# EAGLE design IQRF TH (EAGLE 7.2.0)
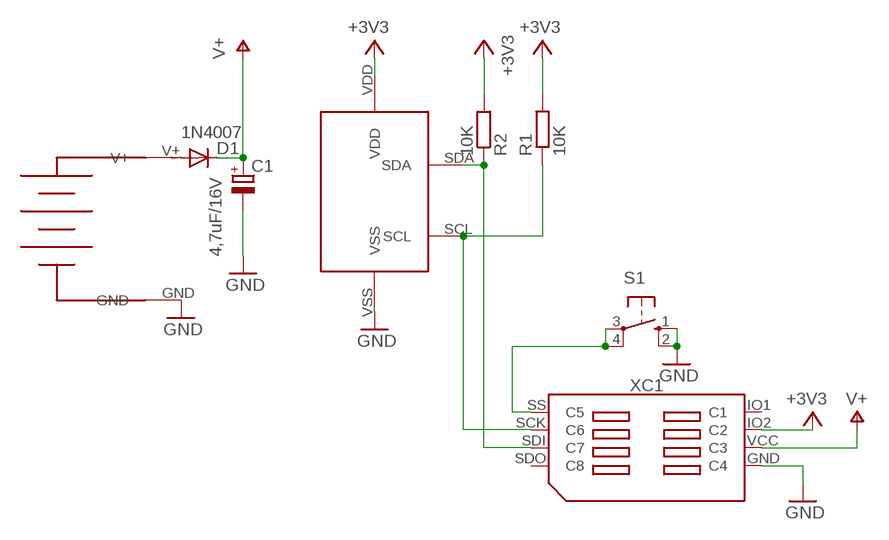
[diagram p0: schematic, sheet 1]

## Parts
3XAA1,5V  3AA  [3AA]
C1  4,7uF/16V  CPOL-EUE2,5-6E  [E2,5-6E]
D1  1N4007  DIODE-DO34-7  [DO34-7]
R1  10K  R-EU_0207/7  [0207/7]
R2  10K  R-EU_0207/7  [0207/7]
S1  10-XX  [B3F-10XX]
U$1  BOB21  [BOB21]
XC1  SIM8X_KON-SIM02  [SIM_02]

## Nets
+3V3: R1.2 R2.2 U$1.VDD XC1.IO2(C2)
GND: 3XAA1,5V.GND C1.- S1.1(S) S1.2(S1) U$1.VSS XC1.GND(C4)
N$1: 3XAA1,5V.V+ D1.A
N$2: R1.1 U$1.SCL XC1.SCK(C6)
N$3: S1.3(P) S1.4(P1) XC1.SS(C5)
N$4: R2.1 U$1.SDA XC1.SDI(C7)
V+: C1.+ D1.C
Unconnected: XC1.IO1(C1) XC1.SDO(C8) XC1.VCC(C3)

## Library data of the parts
3XAA1,5V = battery:3AA
C1 = rcl:CPOL-EU: POLARIZED CAPACITOR, European symbol
D1 = diode:DIODE-: DIODE
R1 R2 = rcl:R-EU_: RESISTOR, European symbol
S1 = switch-omron:10-XX: OMRON SWITCH; MPN: B3F-1000; OC_FARNELL: 176432; OC_NEWARK: 36M3542
U$1 = sinserion:BOB21
XC1 = KON-SIM-02_150624:SIM8X_KON-SIM: KON-SIM-02

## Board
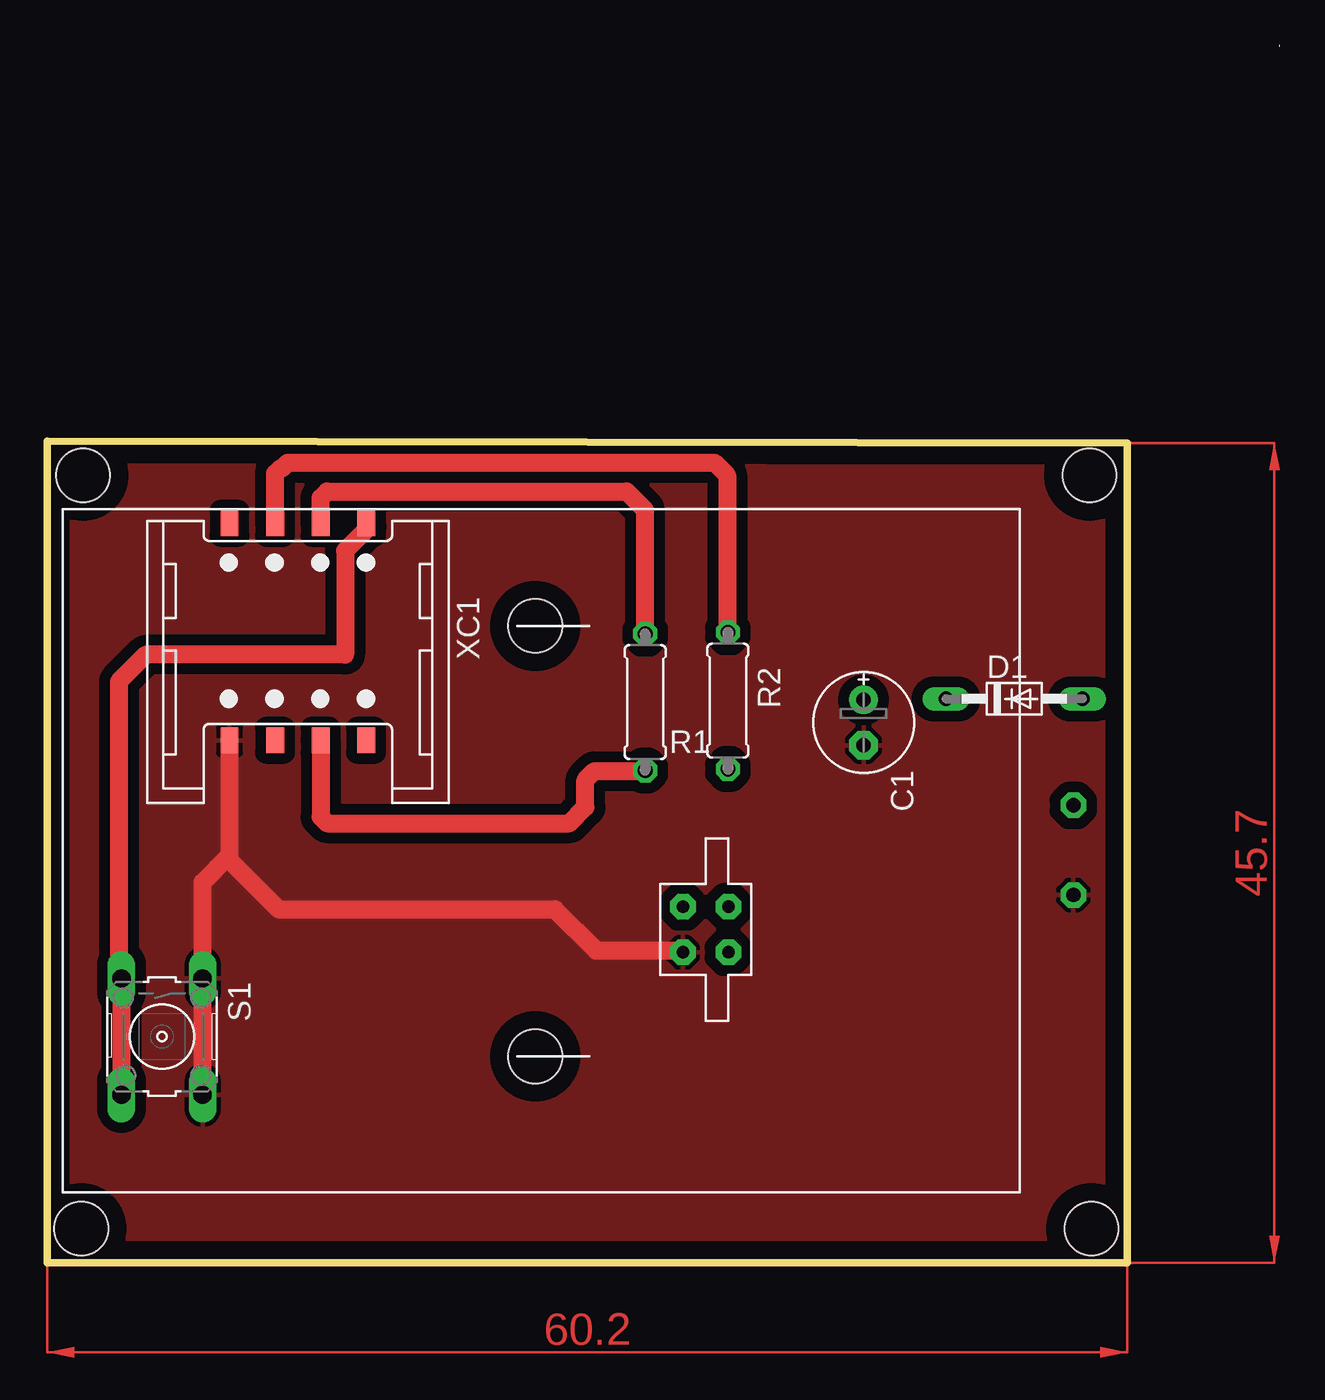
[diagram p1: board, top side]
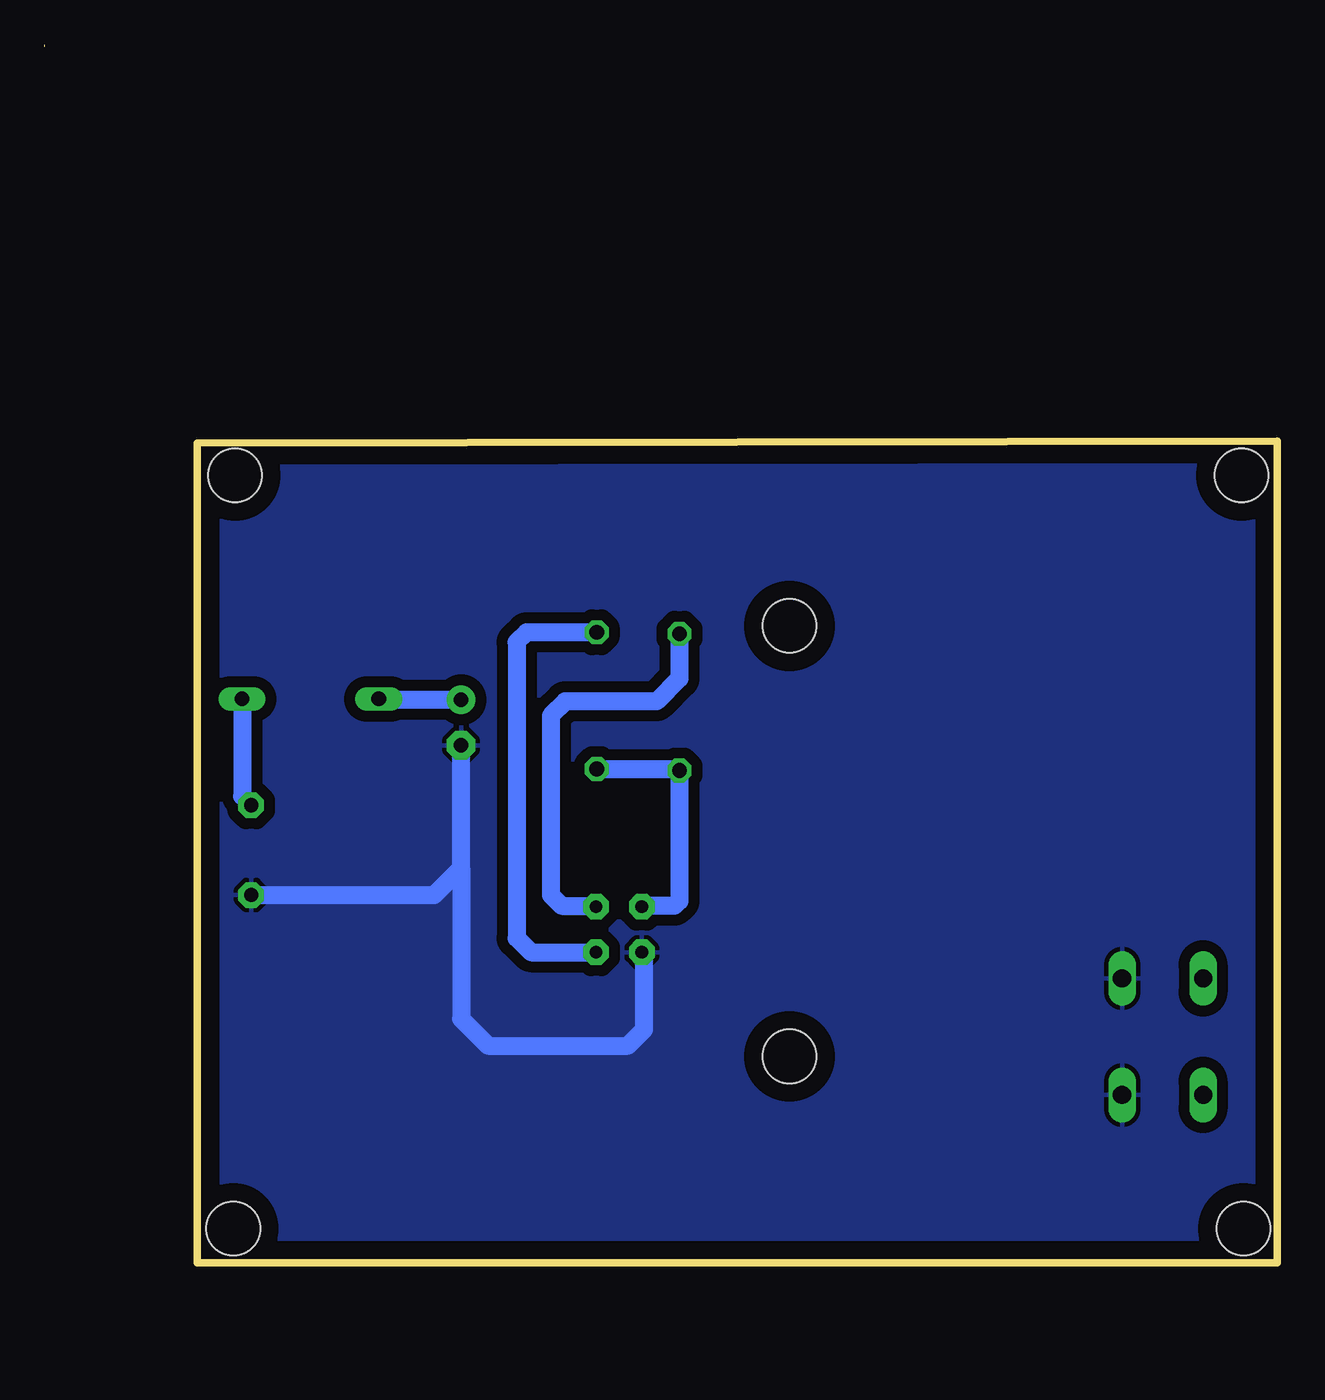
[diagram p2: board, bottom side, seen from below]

Size 68.7 x 67.9 mm. Coordinates in mm from the lower left corner, seen from the top.
Outline: 68.7,67.8 68.7,67.9
Outline: 0,0 60.2,0 60.2,45.7 0,45.8 0,0
Copper layers (1*16): Top 0.035mm / dielectric 1.5mm / Bottom 0.035mm
Design rules "default": minimum track width 10mil, minimum drill 24mil, track to track 8mil, track to pad 8mil, pad to pad 8mil, via to via 8mil, smd to smd 8mil, copper to edge 40mil, drill to drill 8mil, minimum pad ring 10mil, minimum via ring 8mil, stop-mask expansion 4mil, vias tented up to drill 0mil, thermal gap 10mil
Holes 3 mm at 1.9,1.9 58.2,1.9 2,43.9 58.1,43.9

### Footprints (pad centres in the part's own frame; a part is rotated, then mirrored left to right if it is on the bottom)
3AA = drill 0.8 pad 1.422 octagon: GND 36,-5; V+ 36,0 | hole 3: 6,10; 6,-14
E2,5-6E = drill 0.813 pad 1.575: + -1.27,0 | drill 0.813 pad 1.575 octagon: - 1.27,0
DO34-7 = drill 0.813 long: A 3.81,0; C -3.81,0
0207/7 = drill 0.813 octagon: 1 -3.81,0; 2 3.81,0
B3F-10XX = drill 1.016 long: 1 -3.251,2.261; 2 3.251,2.261; 3 -3.251,-2.261; 4 3.251,-2.261
BOB21 = drill 0.7 pad 1.422 octagon: SCL -2.54,1.27; SDA 0,1.27; VDD -2.54,-1.27; VSS 0,-1.27
SIM_02 = smd 1.4 x 1: GND 6.112,-3.81; IO1 6.112,3.81; IO2 6.112,1.27; SCK -5.98,1.27; SDI -5.98,-1.27; SDO -5.98,-3.81; SS -5.98,3.81; VCC 6.112,-1.27

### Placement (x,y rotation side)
3XAA1,5V  21.2,25.5 0 top
C1  45.5,30.11 270 top
D1  53.9,31.44 0 top
R1  33.33,31.25 270 top
R2  37.94,31.33 270 top
S1  6.4,12.6 270 top
U$1  36.7,17.3 270 top
XC1  13.97,35.24 270 top

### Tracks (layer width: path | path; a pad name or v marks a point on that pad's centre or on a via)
+3V3
  Top 1.016: XC1.IO2 15.24,24.86 15.6,24.5 29.1,24.5 30,25.4 30,26.9 30.5,27.4 33.29,27.4 R1.2
  Bottom 1.016: R2.2 33.42,27.52 R1.2 33.33,20.17 33.6,19.9 35.37,19.9 U$1.VDD
GND
  Top 1.016: XC1.GND 10.16,22.7 | 10.16,22.7 10.16,22.44 12.9,19.7 28.3,19.7 30.6,17.4 35.33,17.4 U$1.VSS | S1.1 S1.2 8.66,21.2 10.16,22.7
  Bottom 1.016: 3XAA1,5V.GND 47,20.5 45.5,22 | 45.5,22 C1.- | 45.5,22 45.5,13.6 44,12.1 36.2,12.1 35.3,13 35.3,17.17 U$1.VSS
  pour Bottom (isolate 0.61): 0.8,45.2 59.3,45.2 59.3,0.8 0.6,0.8 0.6,45.1
  pour Top (isolate 0.61): 1,44.4 1,45.2 59.4,45.2 59.4,44.1 59.3,44.1 59.3,0.8 0.7,0.8 0.7,44.6
N$1
  Bottom 1.016: D1.A 57.71,26.01 3XAA1,5V.V+
N$2
  Top 1.016: XC1.SCK 15.24,42.64 15.6,43 32.3,43 33.3,42 33.3,35.09 R1.1
  Bottom 1.016: R1.1 33.33,32.57 34.6,31.3 39.7,31.3 40.5,30.5 40.5,20.5 39.9,19.9 38.03,19.9 U$1.SCL
N$3
  Top 1.016: XC1.SS 17.78,40.88 16.6,39.7 16.6,33.9 5.5,33.9 4,32.4 4,15.99 S1.3 S1.4
N$4
  Top 1.016: XC1.SDI 12.7,44 13,44.3 13.1,44.3 13.4,44.6 37.2,44.6 37.9,43.9 37.9,35.19 R2.1
  Bottom 1.016: R2.1 41.86,35.14 42.4,34.6 42.4,18.1 41.6,17.3 U$1.SDA
V+
  Bottom 1.016: C1.+ 50.03,31.38 D1.C
(copper drawn outside any net)
  shapes: Top area x2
